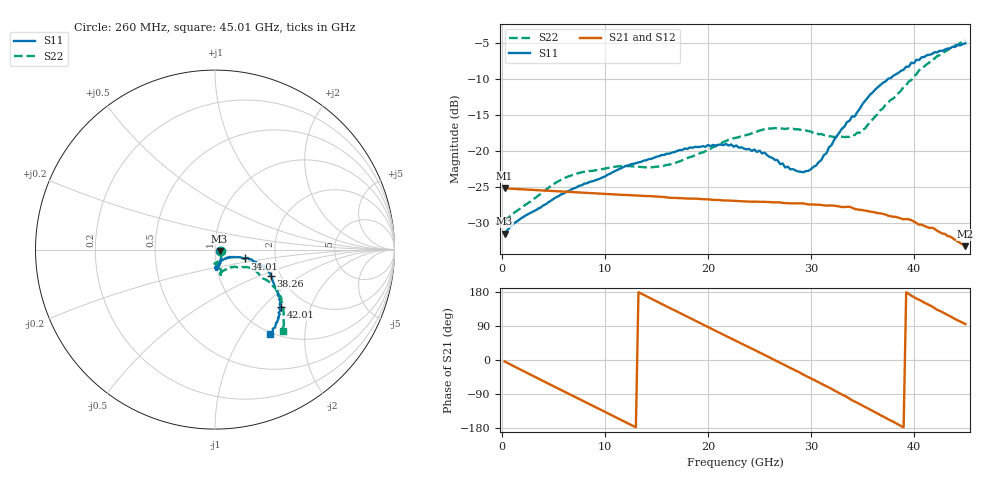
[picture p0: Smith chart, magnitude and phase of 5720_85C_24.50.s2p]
! Device:  ADRF5720
! Description: 0.5dB LSB GaAs MMIC 6-bit Digital Attenuator
! Frequency:  0.000009 -  40 GHz
! Ports:
!	RF1	= Port 1
!	RF2	= Port 2
! Vdd:  3.3 Volt
! Vss:  -3.3 Volt
! Control:  0/3.3 Volt
! State:  24.50 dB attenuation
! Data:  The device was measured using G-S-G Probes on a matrix board.
!  Data was collected using an calibrated 4 port network analyzer.
!  The reference plane for this measurement is at the launchers.
! Note:  Analog Devices supplies this data as a sample of measured data
!  for this product.  Your particular data for this product may vary.
!  Data was taken at 85 degrees C.
!  Analog Devices reserves the right to change this data at anytime.
# GHZ S DB R 45.0
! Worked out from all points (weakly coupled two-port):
!   180 points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, 260 MHz to 45.01 GHz, reference 45 ohm
!   highest |S21| = -25.17 dB at 260 MHz (marker M1); lowest = -33.2 dB at 45.01 GHz (marker M2)
!   lowest |S11| = -31.5 dB at 260 MHz (marker M3), VSWR 1.05, Z = 47.3 - j0.763 ohm
!   |S11| at or under -10 dB: start of sweep to 37.45 GHz
!   |S22| runs from -29.9 to -4.6 dB; largest |S21 - S12| = 0.00034
!   S11 on the Smith chart (normalised r, x): 260 MHz: 1.05, -0.02; 34.01 GHz: 1.40, -0.14; 38.26 GHz: 1.77, -0.59; 42.01 GHz: 1.52, -1.28; 45.01 GHz: 0.97, -1.34
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0.26  -31.47 -17.6  -25.17 -3.8  -25.16 -3.8  -29.91 -15.9
1.76  -29.44 -6.5  -25.29 -24.8  -25.28 -24.7  -27.99 -19.3
5.01  -26.64 -38.9  -25.54 -69.1  -25.52 -69.1  -24.59 -63.1
7.76  -24.74 -53.2  -25.76 -106.4  -25.75 -106.3  -22.93 -80.4
11.51  -22.40 -67.5  -26.06 -157.2  -26.05 -157.1  -22.06 -92.4
15.26  -20.69 -75.6  -26.32 151.4  -26.31 151.5  -22.12 -87.7
18.26  -19.47 -81.3  -26.59 111.0  -26.58 111.1  -20.82 -78.8
22.76  -19.20 -86.8  -26.93 50.0  -26.92 50.2  -18.12 -74.3
25.51  -20.19 -85.7  -27.05 13.2  -27.03 13.4  -16.91 -77.4
28.01  -22.53 -74.3  -27.26 -20.9  -27.25 -20.6  -16.92 -78.2
29.26  -22.93 -54.4  -27.26 -38.3  -27.25 -38.0  -17.04 -78.2
30.26  -22.18 -41.7  -27.41 -51.8  -27.39 -51.6  -17.48 -77.2
31.01  -21.24 -28.8  -27.49 -62.5  -27.47 -62.2  -17.59 -74.2
32.26  -18.42 -20.9  -27.58 -80.0  -27.56 -79.7  -18.02 -67.7
34.01  -15.13 -16.4  -27.87 -106.3  -27.85 -106.1  -17.76 -52.1
34.26  -15.18 -17.6  -28.03 -109.9  -28.02 -109.6  -17.75 -49.1
35.26  -13.00 -17.0  -28.26 -123.6  -28.25 -123.3  -16.84 -41.5
37.76  -9.81 -22.3  -29.06 -159.8  -29.05 -159.4  -12.85 -27.8
38.26  -9.29 -25.3  -29.14 -166.8  -29.11 -166.5  -12.33 -27.2
40.51  -7.31 -35.9  -30.23 159.0  -30.19 159.5  -8.75 -30.9
42.01  -6.21 -41.0  -30.80 136.9  -30.78 137.3  -7.10 -35.1
45.01  -4.98 -57.0  -33.22 94.8  -33.19 95.1  -4.58 -50.4
